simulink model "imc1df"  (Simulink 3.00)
settings: Solver=ode45  SolverMode=SingleTasking  StartTime=0.0  StopTime=50  MaxStep=st_size  RelTol=1e-5  AbsTol=1e-6
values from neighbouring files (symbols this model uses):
  d_through_p = get(MAIN_MENU(19),'Value')    [cback.m]    (also in imcmenu.m = 0)
  Disturb = Setpoint    [mimo_MSF1DF_sim.m]    (also in mimo_MSF2DF_sim.m)
  Satlb = temp1    [cback.m]    (also in imcmenu.m = str2num(satlbs))
  Satub = temp1    [cback.m]    (also in imcmenu.m = str2num(satubs))
  Setpoint = zeros(1,n)    [mimo_MSF1DF_sim.m]    (also in mimo_MSF2DF_sim.m)
undefined symbols (not defined in the file or in its folder): denCs, denMs, denPd, denPs, numCs, numMs, numPd, numPs
libraries: MIMO_lib x2

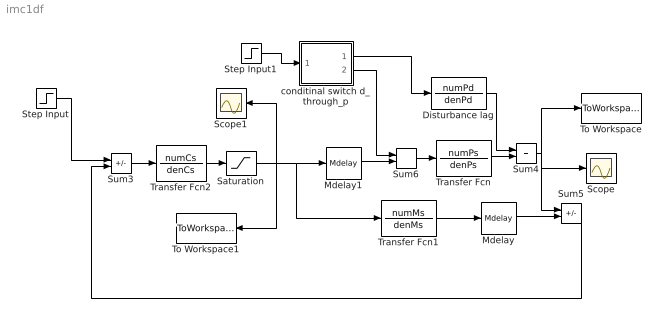
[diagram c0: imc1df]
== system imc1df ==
  Disturbance lag : TransferFcn  Numerator=numPd  Denominator=denPd
  Mdelay : MIMO_lib/Mdelay  Mdelay=Mdelay
  Mdelay1 : MIMO_lib/Mdelay  Mdelay=Pdelay
  Saturation : Saturate  UpperLimit=Satub  LowerLimit=Satlb
  Scope : Scope
  Scope1 : Scope
  Step Input : Step  Time=0  Before=0  After=Setpoint  SampleTime=0
  Step Input1 : Step  Time=0  Before=0  After=Disturb  SampleTime=0
  Sum3 : Sum  Inputs=+-  SaturateOnIntegerOverflow=on
  Sum4 : Sum  Inputs=++  SaturateOnIntegerOverflow=on
  Sum5 : Sum  Inputs=+-  SaturateOnIntegerOverflow=on
  Sum6 : Sum  Inputs=++  SaturateOnIntegerOverflow=on
  To Workspace : ToWorkspace  VariableName=simout  SampleTime=-1  SaveFormat=Matrix
  To Workspace1 : ToWorkspace  VariableName=effort  SampleTime=-1  SaveFormat=Matrix
  Transfer Fcn : TransferFcn  Numerator=numPs  Denominator=denPs
  Transfer Fcn1 : TransferFcn  Numerator=numMs  Denominator=denMs
  Transfer Fcn2 : TransferFcn  Numerator=numCs  Denominator=denCs
  conditinal switch d_through_p : Subsystem  Description=pass input signal through out1 if condition is true.
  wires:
  Sum3/1 -> Transfer Fcn2/1
  Transfer Fcn2/1 -> Saturation/1
  Step Input/1 -> Sum3/1
  Sum5/1 -> Sum3/2
  Sum6/1 -> Transfer Fcn/1
  Transfer Fcn/1 -> Sum4/2
  Disturbance lag/1 -> Sum4/1
  conditinal switch d_through_p/2(Out1) -> Sum6/1
  conditinal switch d_through_p/1(Out2) -> Disturbance lag/1
  Step Input1/1 -> conditinal switch d_through_p/1(In)
  Saturation/1 -> Scope1/1, To Workspace1/1, Mdelay1/1, Transfer Fcn1/1
  Transfer Fcn1/1 -> Mdelay/1
  Mdelay/1 -> Sum5/2
  Sum4/1 -> Sum5/1, Scope/1, To Workspace/1
  Mdelay1/1 -> Sum6/2

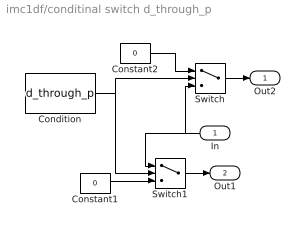
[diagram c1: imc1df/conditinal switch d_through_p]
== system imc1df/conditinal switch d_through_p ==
  In : Inport  Orientation=left  Port=1  PortWidth=-1  SampleTime=-1  DataType=auto
  Condition : Constant  Value=d_through_p
  Constant1 : Constant  Value=0
  Constant2 : Constant  Value=0
  Switch : Switch  Threshold=1
  Switch1 : Switch  Threshold=1
  Out2 : Outport  Port=1  InitialOutput=0
  Out1 : Outport  Port=2  InitialOutput=0
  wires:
  In/1 -> Switch/3, Switch1/1
  Condition/1 -> Switch1/2, Switch/2
  Constant1/1 -> Switch1/3
  Constant2/1 -> Switch/1
  Switch/1 -> Out2/1
  Switch1/1 -> Out1/1
